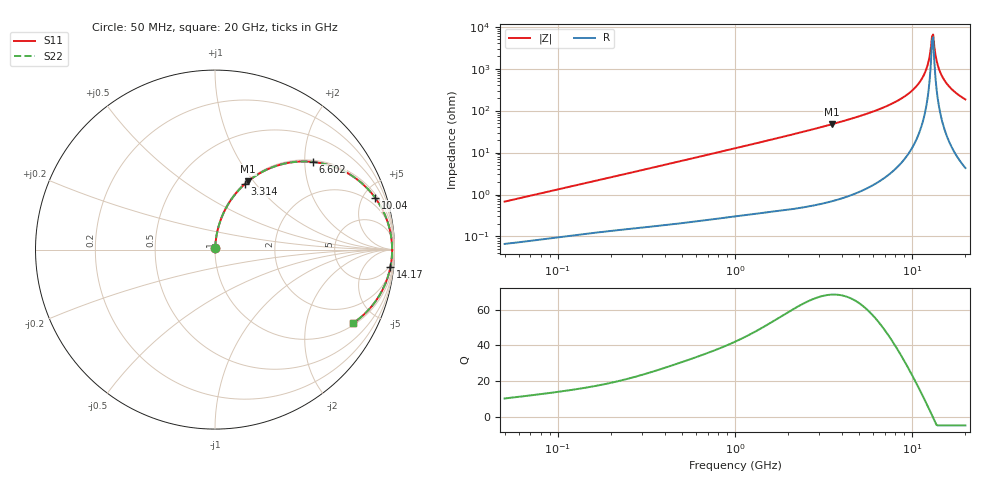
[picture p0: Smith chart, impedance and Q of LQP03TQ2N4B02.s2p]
!Murata Part Number: LQP03TQ2N4B02
!These Parameters are Measured in Series Mode Connection
!  o--[Z]--o
!Port1  Port2
!  o-------o
!Freq. Start=50[MHz] Stop=20[GHz], 401[Steps]
# Hz S RI R 50
!Freq.(Hz) S11(Real) S11(Imag) S21(Real) S21(Imag) S12(Real) S12(Imag) S22(Real) S22(Imag)
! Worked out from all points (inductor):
!   401 points, 50 MHz to 20 GHz, reference 50 ohm
!   read as one part in series: L = 2.13 nH near 51.52 MHz
!   highest Q = 68.5 at 3.519 GHz (marker M1), where L = 2.13 nH
!   self-resonance near 12.95 GHz
!   S11 on the Smith chart (normalised r, x): 50 MHz: 1.00, +0.01; 3.314 GHz: 1.01, +0.88; 6.602 GHz: 1.04, +2.20; 10.04 GHz: 1.27, +6.07; 14.17 GHz: 4, -20; 20 GHz: 1.09, -3.70
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5e7  0.000709 0.00673  0.9993 -0.00673  0.9993 -0.00673  0.000709 0.00673
1.364002e8  0.00144 0.0177  0.9986 -0.0177  0.9986 -0.0177  0.00144 0.0177
3.721004e8  0.00402 0.0471  0.996 -0.0471  0.996 -0.0471  0.00402 0.0471
1e9  0.0185 0.1234  0.9815 -0.1234  0.9815 -0.1234  0.0185 0.1234
2.728004e9  0.1154 0.312  0.8846 -0.312  0.8846 -0.312  0.1154 0.312
3.314454e9  0.1659 0.3648  0.8341 -0.3648  0.8341 -0.3648  0.1659 0.3648
3.519108e9  0.1854 0.3814  0.8146 -0.3814  0.8146 -0.3814  0.1854 0.3814
4.81993e9  0.3268 0.4614  0.6732 -0.4614  0.6732 -0.4614  0.3268 0.4614
6.601595e9  0.5467 0.4883  0.4533 -0.4883  0.4533 -0.4883  0.5467 0.4883
7.442007e9  0.6482 0.4665  0.3518 -0.4665  0.3518 -0.4665  0.6482 0.4665
1.004137e10  0.8922 0.2891  0.1078 -0.2891  0.1078 -0.2891  0.8922 0.2891
1.098561e10  0.9438 0.2002  0.0562 -0.2002  0.0562 -0.2002  0.9438 0.2002
1.183995e10  0.9725 0.1169  0.0275 -0.1169  0.0275 -0.1169  0.9725 0.1169
1.220001e10  0.9798 0.082  0.0202 -0.082  0.0202 -0.082  0.9798 0.082
1.276073e10  0.9859 0.0286  0.0141 -0.0286  0.0141 -0.0286  0.9859 0.0286
1.295331e10  0.9867 0.0106  0.0133 -0.0106  0.0133 -0.0106  0.9867 0.0106
1.334722e10  0.9862 -0.0254  0.0138 0.0254  0.0138 0.0254  0.9862 -0.0254
1.375312e10  0.9832 -0.0612  0.0168 0.0612  0.0168 0.0612  0.9832 -0.0612
1.417136e10  0.9775 -0.0965  0.0225 0.0965  0.0225 0.0965  0.9775 -0.0965
1.504638e10  0.9587 -0.1651  0.0413 0.1651  0.0413 0.1651  0.9587 -0.1651
1.621653e10  0.9226 -0.2444  0.0774 0.2444  0.0774 0.2444  0.9226 -0.2444
2e10  0.7684 -0.4104  0.2316 0.4104  0.2316 0.4104  0.7684 -0.4104
